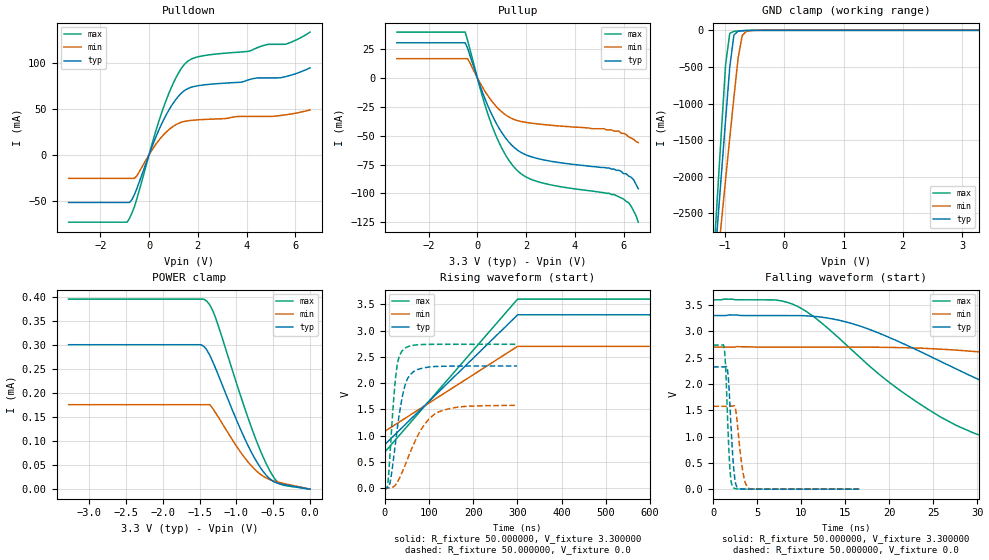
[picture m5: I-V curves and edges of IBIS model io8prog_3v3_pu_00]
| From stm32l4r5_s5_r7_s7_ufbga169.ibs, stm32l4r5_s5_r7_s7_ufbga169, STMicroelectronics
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|   Model io8prog_3v3_pu_00
[Model]  io8prog_3v3_pu_00
Model_type I/O
Polarity   Non-Inverting
Enable   Active-Low
Vinl =   0.990000V
Vinh =   2.310000V
Vmeas =  1.650000V
Cref =   100.000000nF
Rref =   1.000000k
Vref =   3.300000V
C_comp   2.267200pF   2.233100pF   2.322300pF
[Temperature Range]   25.000000   0.125000k   -40.000000
[Pullup Reference]   3.300000V   2.700000V   3.600000V
[Pulldown Reference]   0.0V   0.0V   0.0V
[POWER Clamp Reference]   3.300000V   2.700000V   3.600000V
[GND Clamp Reference]   0.0V   0.0V   0.0V
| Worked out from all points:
|   slope of the pulldown table from 0 to 0.495 V, typ, clamps not added: 15.3 ohm
|   slope of the pullup table from 0 to 0.495 V, typ, clamps not added: 18.1 ohm
|   GND clamp passes 1 mA (typ) near -0.58 V on its own axis
|   rising waveform, R_fixture 50.000000, V_fixture 3.300000: 20-80 % time 180ns typ, 180ns min, 180ns max; typ from 0.832 V to 3.3 V
|   rising waveform, R_fixture 50.000000, V_fixture 0.0: 20-80 % time 24.3ns typ, 54.5ns min, 14.6ns max; typ from 0.001 V to 2.33 V
|   falling waveform, R_fixture 50.000000, V_fixture 3.300000: 20-80 % time 21ns typ, 41.5ns min, 13.7ns max; typ from 3.3 V to 0.832 V
|   falling waveform, R_fixture 50.000000, V_fixture 0.0: 20-80 % time 474ps typ, 656ps min, 393ps max; typ from 2.33 V to 0.001 V
[Pulldown]
|Voltage   I(typ)   I(min)   I(max)
-3.3V     -51.86mA   -25.67mA   -73.32mA
-900mV    -51.86mA   -25.67mA   -73.32mA
-700mV    -48.68mA   -25.67mA   -63.27mA
-500mV    -36.68mA   -22.92mA   -47.9mA
200mV     14.09mA    8.363mA    18.97mA
700mV     43.2mA     24.54mA    59.15mA
1.2V      63.38mA    34mA       88.53mA
1.6V      72.01mA    36.89mA    101.8mA
4.1V      81.56mA    41.59mA    112.4mA
4.9V      83.55mA    41.59mA    120mA
5.6V      84.89mA    43.33mA    120.1mA
6.6V      94.39mA    48.68mA    133.3mA
[Pullup]
|Voltage   I(typ)   I(min)   I(max)
-3.3V     30.51mA    16.73mA    39.78mA
-500mV    30.51mA    16.73mA    39.78mA
-400mV    25.73mA    16.73mA    32.44mA
200mV     -11.99mA   -7.69mA    -15.6mA
500mV     -27.53mA   -17.49mA   -35.6mA
1V        -47.29mA   -29.37mA   -60.81mA
1.5V      -60.05mA   -35.95mA   -77.15mA
1.9V      -65.76mA   -38.13mA   -84.63mA
2.6V      -70.47mA   -40.14mA   -90.6mA
5.6V      -79mA      -46mA      -101mA
6.2V      -85mA      -51mA      -108mA
6.6V      -96mA      -56mA      -125mA
[GND_clamp]
|Voltage   I(typ)   I(min)   I(max)
-3.3V     -9.456A    -9.706A    -9.779A
-1.2V     -3.441A    -3.76A     -3.218A
-1.13V    -2.694A    -3.182A    -2.288A
-1.06V    -1.951A    -2.607A    -1.365A
-990mV    -1.216A    -2.035A    -464.9mA
-920mV    -500mA     -1.468A    -40.15mA
-850mV    -63.51mA   -913mA     -13.79mA
-780mV    -11.84mA   -384.3mA   -8.858mA
-710mV    -4.78mA    -70.26mA   -5.228mA
-640mV    -2.25mA    -14.29mA   -2.447mA
-430mV    -27.1uA    -149uA     -11.19uA
3.28V     0A         0A         0A
[POWER_clamp]
|Voltage   I(typ)   I(min)   I(max)
-3.28V    301.3uA    176.2uA    396.6uA
-1.48V    301.3uA    176.2uA    396.6uA
-1.4V     290uA      176.2uA    391.9uA
-1.36V    278.9uA    176.2uA    384uA
-1.28V    250.9uA    158.7uA    356.2uA
-1V       144.8uA    89.98uA    221.7uA
-840mV    90.38uA    56.36uA    147.8uA
-680mV    46.32uA    31.78uA    82.44uA
-560mV    23.38uA    20.73uA    42.33uA
-480mV    14.66uA    16.5uA     21.94uA
-400mV    10.77uA    13.43uA    10.23uA
0V        0A         0A         0A
[Ramp]
| variable   typ   min   max
dV/dt_r  1.39450/24.32029n   0.94482/54.54234n   1.64288/14.56534n
dV/dt_f  1.48066/21.06490n   0.97008/44.49579n   1.74725/13.65133n
R_load = 50.000000
[Rising Waveform]
R_fixture= 50.000000
V_fixture= 3.300000
V_fixture_min= 2.700000
V_fixture_max= 3.600000
|time   V(typ)   V(min)   V(max)
0s        832.2mV    1.083V     687.9mV
300.3ns   3.3V       2.7V       3.6V
600.6ns   3.3V       2.7V       3.6V
29.73us   3.3V       2.7V       3.6V
[Rising Waveform]
R_fixture= 50.000000
V_fixture= 0.0
V_fixture_min= 0.0
V_fixture_max= 0.0
|time   V(typ)   V(min)   V(max)
0s        929.1uV    1.395mV    658.7uV
7.207ns   6.479mV    4.346mV    119.8mV
12.61ns   142.1mV    5.612mV    767.6mV
19.82ns   573.9mV    27.38mV    1.677V
27.63ns   1.104V     104.5mV    2.328V
41.44ns   1.817V     349.8mV    2.637V
64.86ns   2.22V      832.4mV    2.72V
88.89ns   2.292V     1.204V     2.736V
122.5ns   2.319V     1.455V     2.739V
299.1ns   2.325V     1.576V     2.739V
[Falling Waveform]
R_fixture= 50.000000
V_fixture= 3.300000
V_fixture_min= 2.700000
V_fixture_max= 3.600000
|time   V(typ)   V(min)   V(max)
0s        3.3V       2.7V       3.6V
9.61ns    3.3V       2.7V       3.473V
15.62ns   3.157V     2.7V       2.667V
24.62ns   2.527V     2.672V     1.495V
29.73ns   2.117V     2.617V     1.058V
33.63ns   1.831V     2.557V     907.2mV
46.55ns   1.158V     2.272V     764.1mV
60.06ns   970.6mV    1.923V     721.1mV
93.69ns   862.2mV    1.287V     693.7mV
149.5ns   832.2mV    1.083V     687.9mV
[Falling Waveform]
R_fixture= 50.000000
V_fixture= 0.0
V_fixture_min= 0.0
V_fixture_max= 0.0
|time   V(typ)   V(min)   V(max)
0s        2.325V     1.576V     2.739V
1.235ns   2.325V     1.576V     2.705V
1.435ns   2.33V      1.576V     2.254V
1.702ns   2.151V     1.576V     1.063V
1.969ns   1.384V     1.576V     247.4mV
2.302ns   455.4mV    1.585V     27.13mV
2.703ns   41.82mV    1.315V     5.034mV
3.403ns   2.182mV    304mV      3.038mV
4.037ns   1.17mV     17.22mV    3.006mV
16.62ns   929.1uV    1.395mV    658.7uV
